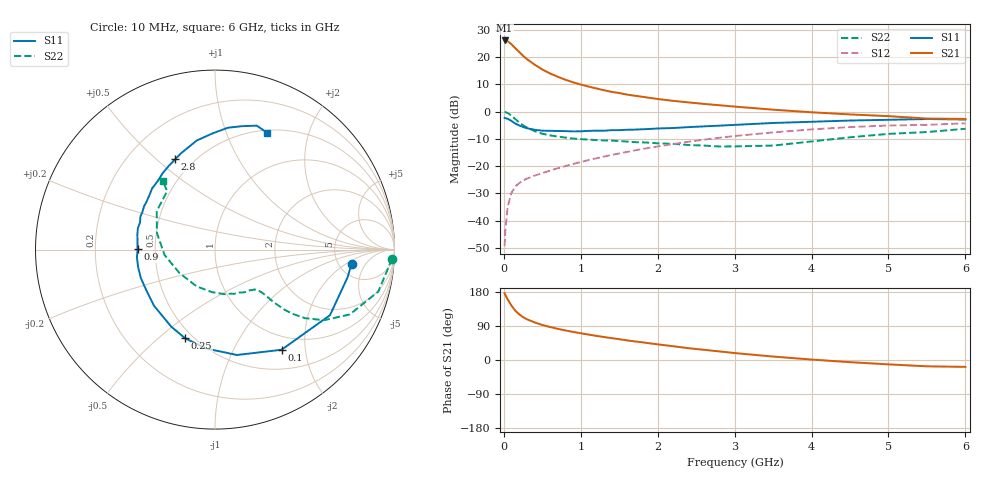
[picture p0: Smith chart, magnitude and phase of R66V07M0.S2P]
! SIEMENS Small Signal Semiconductors
! BFR193
! Si NPN RF Bipolar Junction Transistor in SOT23
! VCE = 6 V  IC = 7 mA
! Common Emitter S-Parameters:  May  1996
# GHz  S  MA  R  50
!  f  S11  S21  S12  S22
! GHz  MAG  ANG  MAG  ANG  MAG  ANG  MAG  ANG
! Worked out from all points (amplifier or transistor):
!   36 points, 10 MHz to 6 GHz, reference 50 ohm
!   highest |S21| = 26.0 dB at 10 MHz (marker M1)
!   |S21| within 3 dB of that: start of sweep to 155.4 MHz
!   unconditionally stable (mu >= 1): 836.1 MHz to 2.019 GHz
!   at 250 MHz: K = 0.52, MSG = 22.8 dB, |S12| = -25.3 dB
!   at 1.4 GHz: K = 1.05, MAG = 10.3 dB, |S12| = -16.0 dB
!   at 6 GHz: K = 0.95, MSG = 0.8 dB, |S12| = -4.3 dB
!   lowest NFmin = 1.20 dB at 450 MHz
!   S11 on the Smith chart (normalised r, x): 10 MHz: 6.51, -2.51; 100 MHz: 0.78, -1.58; 250 MHz: 0.45, -0.62; 900 MHz: 0.40, +0.00; 2.8 GHz: 0.40, +0.58; 6 GHz: 0.53, +1.41
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0.01  0.7647 -6.0  20.06 176.0  0.0034 83.1  0.9875 -2.9
0.02  0.7544 -11.9  19.88 171.6  0.0069 86.7  0.9713 -5.9
0.05  0.7376 -29.7  19.4 159.9  0.018 74.5  0.9395 -14.4
0.1  0.67 -56.4  17.03 143.3  0.0325 65.2  0.8334 -25.7
0.15  0.5998 -78.2  14.45 129.9  0.0426 57.9  0.724 -32.9
0.2  0.5537 -94.9  12.34 120.4  0.0486 54.1  0.6306 -37.3
0.25  0.5216 -108.5  10.48 113.1  0.0544 52.3  0.559 -39.7
0.3  0.4934 -119.7  9.12 107.5  0.0588 51.9  0.5103 -40.9
0.4  0.4621 -137.3  7.235 99.2  0.0667 52.3  0.4368 -41.9
0.5  0.4447 -149.2  5.893 92.5  0.0742 53.8  0.3911 -42.1
0.6  0.4426 -159.0  4.984 87.1  0.0826 55.2  0.3654 -42.3
0.7  0.4395 -167.0  4.34 82.3  0.091 56.4  0.3479 -42.7
0.9  0.4314 179.8  3.436 74.1  0.1095 58.8  0.3193 -44.3
1.1  0.4407 169.1  2.869 67.2  0.1288 60.0  0.3059 -47.5
1.3  0.4441 160.2  2.458 60.7  0.149 60.4  0.2949 -50.9
1.6  0.463 148.7  2.043 51.8  0.1814 59.9  0.2815 -58.2
2.2  0.498 129.7  1.569 36.4  0.2532 56.0  0.2552 -77.2
2.8  0.5503 113.7  1.304 22.7  0.3299 49.2  0.2287 -105.0
3.5  0.6163 99.5  1.08 9.1  0.4139 39.0  0.2374 -146.7
4.5  0.6831 83.9  0.884 -5.7  0.5179 23.4  0.3368 164.0
5.5  0.7286 71.4  0.742 -16.7  0.5693 7.1  0.4203 129.4
6  0.7132 65.9  0.73 -18.1  0.6076 2.3  0.4819 127.1
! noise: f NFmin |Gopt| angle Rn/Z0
0.45  1.2  0.24  125  0.12
0.9  1.25  0.36  154  0.11
1.8  2  0.55  -156  0.13
